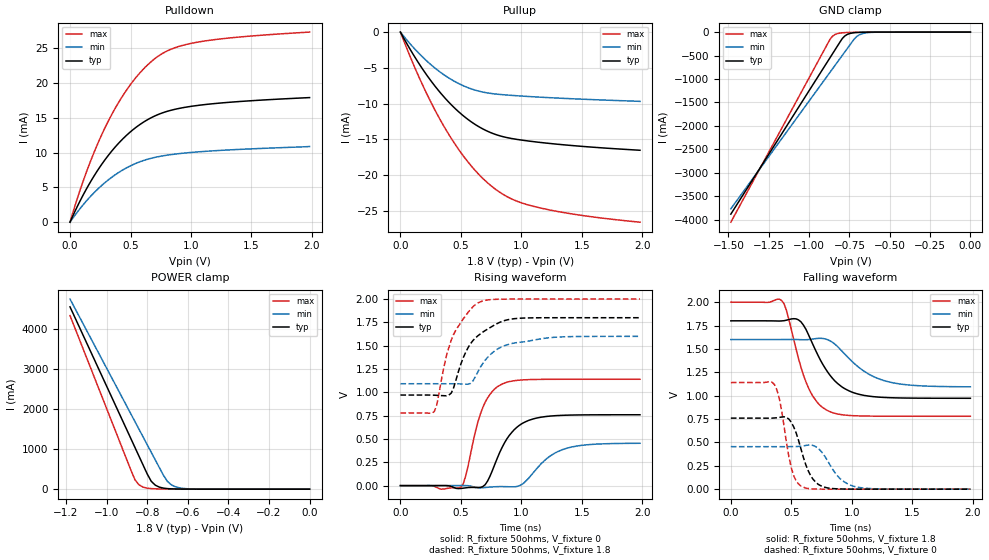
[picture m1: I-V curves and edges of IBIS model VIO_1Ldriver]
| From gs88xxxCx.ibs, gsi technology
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|  signals   DQA1-DQA9, DQB1-DQB9, DQC1-DQC9, DQD1-DQD9
[Model]   VIO_1Ldriver
Model_type   I/O
Polarity   Non-Inverting
Vinl  =   0.75v
Vinh  =   1.75v
Vmeas =   1.25v
Cref  =   0.0pF
Rref  =   50
Vref  =   1.25v
|  variable   typ   min   max
C_comp   3.0pF   2.5pF   3.5pF
|  variable   typ   min   max
[Temperature Range]   50   0   100
|  variable   typ   min   max
[Voltage Range]   1.8   1.6   2.0
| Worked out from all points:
|   slope of the pulldown table from 0 to 0.27 V, typ, clamps not added: 31.7 ohm
|   slope of the pullup table from 0 to 0.27 V, typ, clamps not added: 37.4 ohm
|   GND clamp passes 1 mA (typ) near -0.61 V on its own axis
|   POWER clamp passes 1 mA (typ) near -0.59 V on its own axis
|   rising waveform, R_fixture 50ohms, V_fixture 0: 20-80 % time 191ps typ, 231ps min, 146ps max; typ from 0 V to 0.76 V
|   rising waveform, R_fixture 50ohms, V_fixture 1.8: 20-80 % time 209ps typ, 227ps min, 180ps max; typ from 0.971 V to 1.8 V
|   falling waveform, R_fixture 50ohms, V_fixture 1.8: 20-80 % time 228ps typ, 292ps min, 174ps max; typ from 1.8 V to 0.972 V
|   falling waveform, R_fixture 50ohms, V_fixture 0: 20-80 % time 119ps typ, 153ps min, 90.8ps max; typ from 0.76 V to 0 V
[Pulldown]
| voltage   typ   min   max
0V        -278.2pA   -874.6pA   -161.2pA
80mV      2.946mA    1.887mA    4.45mA
160mV     5.522mA    3.527mA    8.34mA
240mV     7.759mA    4.936mA    11.73mA
320mV     9.684mA    6.13mA     14.66mA
400mV     11.32mA    7.126mA    17.18mA
500mV     13mA       8.11mA     19.8mA
600mV     14.31mA    8.828mA    21.9mA
700mV     15.27mA    9.314mA    23.5mA
840mV     16.12mA    9.732mA    24.91mA
1.06V     16.8mA     10.11mA    25.91mA
1.98V     17.92mA    10.88mA    27.34mA
[Pullup]
| voltage (VDDQ-Vout)   typ   min   max
0V        208.8pA    794.2pA    88.98pA
80mV      -2.401mA   -1.638mA   -3.41mA
180mV     -5.088mA   -3.433mA   -7.281mA
280mV     -7.433mA   -4.953mA   -10.73mA
380mV     -9.443mA   -6.201mA   -13.76mA
560mV     -12.24mA   -7.783mA   -18.19mA
660mV     -13.35mA   -8.306mA   -20.11mA
760mV     -14.15mA   -8.606mA   -21.64mA
920mV     -14.88mA   -8.851mA   -23.34mA
1.14V     -15.4mA    -9.086mA   -24.53mA
1.5V      -15.98mA   -9.381mA   -25.64mA
1.98V     -16.52mA   -9.69mA    -26.58mA
[GND Clamp]
| voltage   typ   min   max
-1.485V   -3.884A    -3.771A    -4.056A
-885mV    -626.9mA   -926.9mA   -247.2mA
-870mV    -545.6mA   -856mA     -153.5mA
-855mV    -464.4mA   -785mA     -89.11mA
-825mV    -301.9mA   -643.2mA   -32.88mA
-795mV    -141.5mA   -501.4mA   -15.38mA
-780mV    -86.61mA   -430.5mA   -11.65mA
-750mV    -32.85mA   -288.8mA   -7.734mA
-705mV    -8.727mA   -95.28mA   -4.834mA
-660mV    -2.907mA   -24.97mA   -2.925mA
-555mV    -316.7uA   -1.176mA   -484.9uA
0V        -278.2pA   -874.6pA   -161.2pA
[POWER Clamp]
| voltage (VDDQ-Vout)   typ   min   max
-1.18V    4.545A     4.74A      4.328A
-880mV    1.258A     1.875A     474.1mA
-860mV    1.039A     1.684A     234.3mA
-840mV    820.4mA    1.493A     107.4mA
-820mV    601.5mA    1.302A     50.64mA
-780mV    197.3mA    920.5mA    14.28mA
-760mV    99.71mA    729.7mA    9.034mA
-720mV    26.23mA    348.2mA    4.898mA
-700mV    13.96mA    192.6mA    3.916mA
-660mV    4.495mA    57.55mA    2.579mA
-560mV    510.5uA    2.941mA    648.3uA
0V        209pA      794.1pA    88.9pA
[Ramp]
| voltage   typ   min   max
dV/dt_r   0.86/129p   0.71/171p   1.10/103p
dV/dt_f   0.86/129p   0.66/166p   1.07/101p
R_load  =   50ohms
[Rising Waveform]
C_fixture =   0.0pF
R_fixture =   50ohms
V_fixture =   0
| Time   V(typ)   V(min)   V(max)
0s        4.693nV    19.34nV    2.031nV
500ps     -30.83mV   651.1uV    -16.88mV
540ps     -23.85mV   440.8uV    106.2mV
620ps     -19.71mV   -19.55mV   581.1mV
680ps     -11.04mV   -23.02mV   834.3mV
840ps     408.6mV    -10.7mV    1.089V
1ns       661.1mV    9.019mV    1.132V
1.12ns    722.5mV    172mV      1.138V
1.38ns    755.2mV    402.4mV    1.14V
1.98ns    759.6mV    453.8mV    1.14V
[Rising Waveform]
C_fixture =   0.0pF
R_fixture =   50ohms
V_fixture =   1.8
V_fixture_min =  1.6
V_fixture_max =  2.0
| Time   V(typ)   V(min)   V(max)
0s        971mV      1.092V     779.2mV
280ps     969.3mV    1.092V     793.5mV
300ps     967.9mV    1.092V     863.1mV
380ps     963mV      1.092V     1.391V
420ps     991.9mV    1.092V     1.559V
540ps     1.431V     1.087V     1.825V
640ps     1.606V     1.219V     1.958V
760ps     1.709V     1.424V     1.995V
920ps     1.786V     1.523V     2V
1.98ns    1.8V       1.6V       2V
[Falling Waveform]
C_fixture =   0.0pF
R_fixture =   50ohms
V_fixture =   1.8
V_fixture_min =  1.6
V_fixture_max =  2.0
| Time   V(typ)   V(min)   V(max)
0s        1.8V       1.6V       2V
420ps     1.799V     1.6V       2.017V
460ps     1.807V     1.6V       1.91V
540ps     1.821V     1.6V       1.492V
620ps     1.711V     1.598V     1.149V
700ps     1.486V     1.61V      953.9mV
800ps     1.253V     1.598V     839.8mV
980ps     1.049V     1.394V     788.2mV
1.26ns    981.3mV    1.163V     780.3mV
1.98ns    971.8mV    1.095V     779.6mV
[Falling Waveform]
C_fixture =   0.0pF
R_fixture =   50ohms
V_fixture =   0
| Time   V(typ)   V(min)   V(max)
0s        759.6mV    454.6mV    1.14V
360ps     761.2mV    454.4mV    1.119V
400ps     767.7mV    454.3mV    973.7mV
500ps     714.8mV    455.3mV    226.8mV
540ps     600.4mV    455.9mV    89.4mV
600ps     338mV      463mV      21.11mV
720ps     53.36mV    438.7mV    1.089mV
900ps     2.558mV    116.1mV    32.75uV
1.02ns    398.8uV    29.63mV    7.894uV
1.98ns    1.493uV    7.149uV    503.7nV
